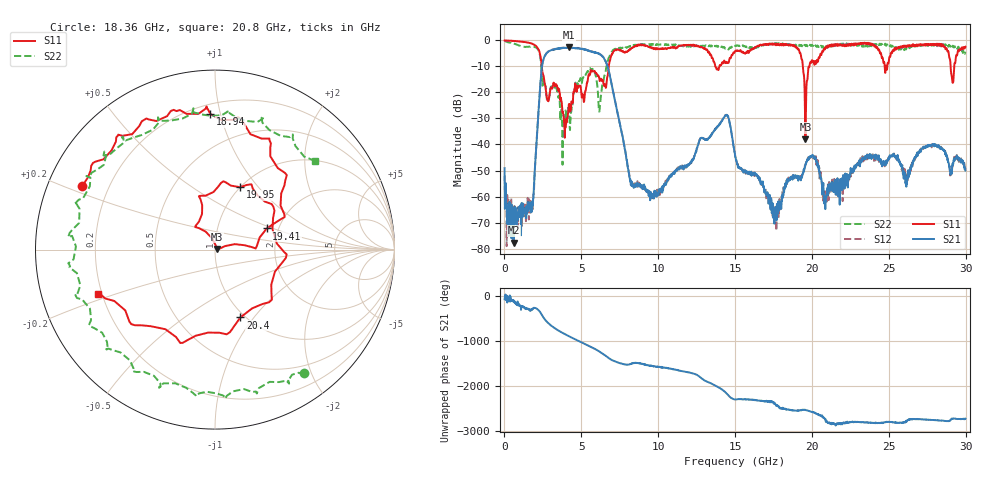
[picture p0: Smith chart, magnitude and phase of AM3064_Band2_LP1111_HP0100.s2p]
# Hz S DB R 50.0
!freq dBS11 angS11 dBS21 angS21 dBS12 angS12 dBS22 angS22
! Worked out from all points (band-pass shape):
!   1600 points, 10 MHz to 29.98 GHz, reference 50 ohm
!   highest |S21| = -2.73 dB at 4.19 GHz (marker M1); lowest = -77.7 dB at 591.1 MHz (marker M2)
!   |S21| within 3 dB of the highest: 2.649 GHz to 6.297 GHz (3.648 GHz wide, 81.6 % of centre)
!   lowest |S11| = -37.9 dB at 19.58 GHz (marker M3), VSWR 1.03, Z = 51.2 + j0.418 ohm
!   |S11| at or under -10 dB: 2.425 GHz to 6.785 GHz (4.36 GHz wide, 94.7 % of centre); 13.71 GHz to 13.98 GHz (268 MHz wide, 1.94 % of centre); 19.41 GHz to 19.84 GHz (427.4 MHz wide, 2.18 % of centre)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
!   |S22| runs from -47.8 to -0.1 dB; largest |S21 - S12| = 0.023
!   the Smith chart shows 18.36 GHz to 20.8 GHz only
!   S11 on the Smith chart (normalised r, x): 18.36 GHz: 0.10, +0.23; 18.94 GHz: 0.26, +0.93; 19.41 GHz: 1.73, +0.45; 19.95 GHz: 1.00, +0.81; 20.4 GHz: 0.95, -0.86; 20.8 GHz: 0.18, -0.18
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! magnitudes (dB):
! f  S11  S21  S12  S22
! 10 MHz  0.0  -49.1  -52.1  -0.1
! 591.1 MHz  -0.2  -77.7  -71.5  -1.2
! 1.791 GHz  -1.2  -65.8  -63.0  -2.4
! 2.597 GHz  -15.8  -6.3  -6.3  -16.1
! 4.19 GHz  -24.5  -2.7  -2.9  -26.7
! 5.015 GHz  -21.1  -3.3  -3.2  -15.9
! 6.627 GHz  -17.2  -8.7  -8.8  -10.2
! 8.276 GHz  -2.9  -54.5  -55.3  -2.1
! 10 GHz  -3.3  -59.6  -58.2  -1.6
! 14.39 GHz  -8.6  -28.8  -28.8  -3.2
! 15 GHz  -4.1  -44.6  -44.2  -2.1
! 17.57 GHz  -1.2  -65.2  -68.5  -1.4
! 18.36 GHz  -1.7  -54.9  -55.3  -1.4
! 18.94 GHz  -2.4  -52.5  -52.7  -1.6
! 19.41 GHz  -10.1  -50.9  -51.0  -1.8
! 19.58 GHz  -37.9  -47.4  -47.8  -2.0
! 19.95 GHz  -8.5  -44.6  -44.9  -2.2
! 19.99 GHz  -7.7  -44.6  -44.7  -1.7
! 20.4 GHz  -7.9  -48.8  -47.8  -2.4
! 20.8 GHz  -3.1  -62.7  -59.8  -2.6
! 25 GHz  -8.3  -45.0  -45.4  -1.6
! 29.98 GHz  -2.5  -50.0  -49.7  -4.3
